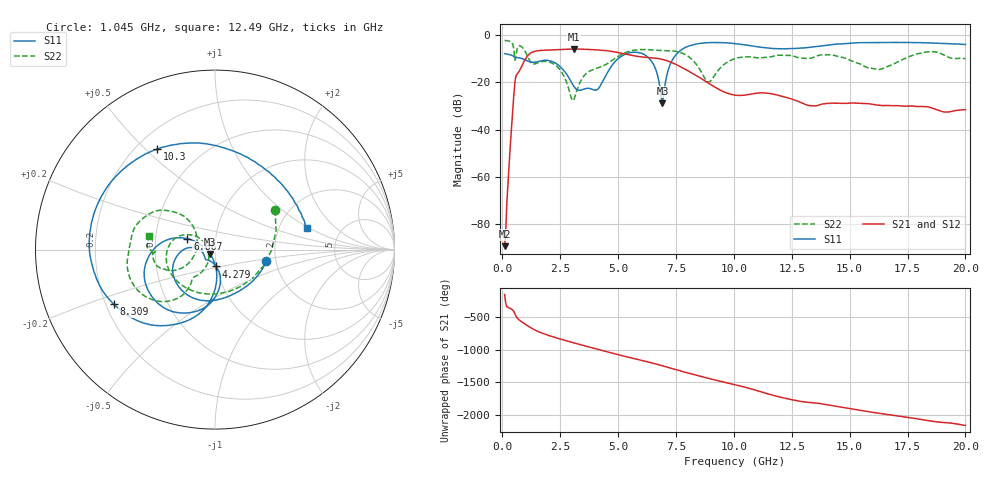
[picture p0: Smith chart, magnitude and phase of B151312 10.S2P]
!  2-Port S-parameters saved by WinCal
! VAR MeasName=S-Parameters (CALIBRATED_DATA) read from VNA (N5244A)
! VAR MeasDate=12/8/2015 5:44:24 PM
! VAR NAME=B151312 10
! VAR FILENAME=B151312 10.S2P
! VAR DATE=12/8/2015 5:44:24 PM
! VAR PHYS_PORTS=1,2
# Hz S DB R 50
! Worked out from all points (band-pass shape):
!   401 points, 100 MHz to 20 GHz, reference 50 ohm
!   highest |S21| = -5.80 dB at 3.085 GHz (marker M1); lowest = -89.4 dB at 100 MHz (marker M2)
!   |S21| within 3 dB of the highest: 1.091 GHz to 5.759 GHz (4.669 GHz wide, 136 % of centre)
!   lowest |S11| = -28.8 dB at 6.916 GHz (marker M3), VSWR 1.08, Z = 47.3 - j2.25 ohm
!   |S11| at or under -10 dB: 889.9 MHz to 4.992 GHz (4.102 GHz wide, 139 % of centre); 6.362 GHz to 7.372 GHz (1.01 GHz wide, 14.7 % of centre)
!   |S22| runs from -27.6 to -2.2 dB; largest |S21 - S12| = 0.0015
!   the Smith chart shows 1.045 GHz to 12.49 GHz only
!   S11 on the Smith chart (normalised r, x): 1.045 GHz: 1.78, -0.24; 4.279 GHz: 0.99, -0.19; 6.667 GHz: 0.73, +0.09; 8.309 GHz: 0.23, -0.24; 10.3 GHz: 0.28, +0.54; 12.49 GHz: 2.86, +0.94
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1e8  -7.80 165.0  -89.35 -162.5  -81.42 95.1  -2.19 169.3
5.4775e8  -9.45 91.8  -19.57 -94.9  -19.57 -94.9  -10.54 112.1
8.4625e8  -9.84 32.2  -13.03 141.0  -13.03 141.0  -4.97 87.7
1.04525e9  -10.67 -12.2  -9.40 93.8  -9.40 93.8  -7.95 33.3
1.54275e9  -11.14 -84.2  -6.53 -4.2  -6.53 -4.2  -11.62 -120.4
2.13975e9  -11.07 -143.3  -6.20 -80.9  -6.20 -80.9  -11.78 175.6
3.085e9  -21.56 -178.8  -5.80 -178.0  -5.80 -178.0  -27.44 -149.9
3.43325e9  -23.10 -145.7  -5.88 148.2  -5.87 148.2  -18.55 -118.8
4.279e9  -20.56 -86.6  -6.32 69.2  -6.32 69.2  -13.25 -126.8
5.52275e9  -7.31 -130.6  -8.38 -42.8  -8.38 -42.9  -6.65 -145.2
6.667e9  -15.64 158.4  -9.77 -142.4  -9.78 -142.5  -6.36 -178.4
6.7665e9  -19.61 158.4  -9.91 -152.3  -9.92 -152.3  -6.40 179.7
6.91575e9  -28.77 -139.3  -10.20 -167.4  -10.22 -167.4  -6.47 176.9
7.41325e9  -9.37 -100.7  -11.95 141.8  -11.94 141.7  -6.69 164.1
8.30875e9  -3.86 -151.9  -16.69 56.1  -16.65 55.8  -11.46 133.8
8.90575e9  -3.11 -179.1  -20.32 1.4  -20.30 1.1  -19.85 170.5
1.005e10  -3.52 131.1  -25.36 -95.3  -25.40 -95.4  -9.84 -161.6
1.029875e10  -3.80 119.8  -25.49 -116.4  -25.52 -116.6  -9.34 -167.0
1.248775e10  -5.59 13.1  -27.00 37.9  -27.01 38.3  -8.58 168.5
1.338325e10  -5.03 -26.3  -29.91 -9.4  -29.86 -8.9  -9.57 172.2
1.67165e10  -3.04 -113.6  -29.81 168.4  -29.62 168.2  -12.90 -177.3
2e10  -3.89 -150.3  -31.60 4.6  -31.62 3.6  -9.93 134.3
